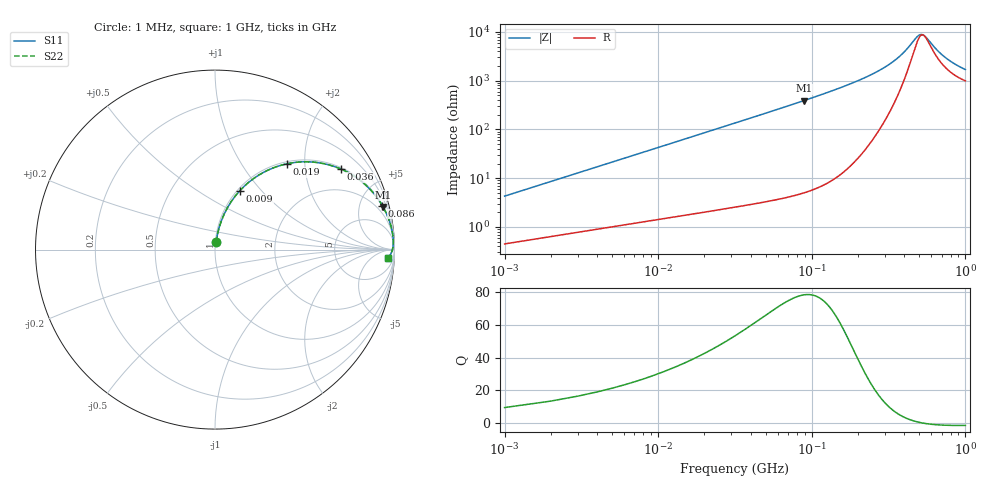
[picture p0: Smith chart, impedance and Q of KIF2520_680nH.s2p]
!version-2
!date-12.2020
!Series
# MHz S RI R 50
!Freq ReS11 ImS11 ReS21 ImS21 ReS12 ImS12 ReS22 ImS22
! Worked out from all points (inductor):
!   1000 points, 1 MHz to 1 GHz, reference 50 ohm
!   read as one part in series: L = 680 nH near 6 MHz
!   highest Q = 78.2 at 89 MHz (marker M1), where L = 701 nH
!   self-resonance near 532.8 MHz
!   S11 on the Smith chart (normalised r, x): 1 MHz: 1.01, +0.09; 9 MHz: 1.03, +0.77; 19 MHz: 1.04, +1.63; 36 MHz: 1.05, +3.09; 86 MHz: 1.10, +7.56; 1 GHz: 21, -27
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1  0.00627 0.0423  0.9937 -0.0423  0.9937 -0.0423  0.00627 0.0423
7  0.0912 0.2687  0.9088 -0.2687  0.9088 -0.2687  0.0912 0.2687
9  0.1375 0.3273  0.8625 -0.3273  0.8625 -0.3273  0.1375 0.3273
13  0.2425 0.4143  0.7575 -0.4143  0.7575 -0.4143  0.2425 0.4143
19  0.4004 0.4781  0.5996 -0.4781  0.5996 -0.4781  0.4004 0.4781
27  0.571 0.4849  0.429 -0.4849  0.429 -0.4849  0.571 0.4849
36  0.7017 0.4487  0.2983 -0.4487  0.2983 -0.4487  0.7017 0.4487
45  0.786 0.4023  0.214 -0.4023  0.214 -0.4023  0.786 0.4023
56  0.8507 0.3492  0.1493 -0.3492  0.1493 -0.3492  0.8507 0.3492
86  0.9318 0.2457  0.0682 -0.2457  0.0682 -0.2457  0.9318 0.2457
89  0.9362 0.2381  0.0638 -0.2381  0.0638 -0.2381  0.9362 0.2381
168  0.9825 0.1222  0.0175 -0.1222  0.0175 -0.1222  0.9825 0.1222
334  0.9933 0.041  0.00671 -0.041  0.00671 -0.041  0.9933 0.041
396  0.9926 0.0252  0.00737 -0.0252  0.00737 -0.0252  0.9926 0.0252
474  0.9906 0.0096  0.00936 -0.0096  0.00936 -0.0096  0.9906 0.0096
501  0.9897 0.00501  0.0103 -0.00501  0.0103 -0.00501  0.9897 0.00501
520  0.989 0.00197  0.011 -0.00197  0.011 -0.00197  0.989 0.00197
541  0.9882 -0.00122  0.0118 0.00122  0.0118 0.00122  0.9882 -0.00122
667  0.9826 -0.0174  0.0174 0.0174  0.0174 0.0174  0.9826 -0.0174
743  0.9788 -0.0252  0.0212 0.0252  0.0212 0.0252  0.9788 -0.0252
834  0.9739 -0.0332  0.0261 0.0332  0.0261 0.0332  0.9739 -0.0332
1000  0.9645 -0.0445  0.0355 0.0445  0.0355 0.0445  0.9645 -0.0445
